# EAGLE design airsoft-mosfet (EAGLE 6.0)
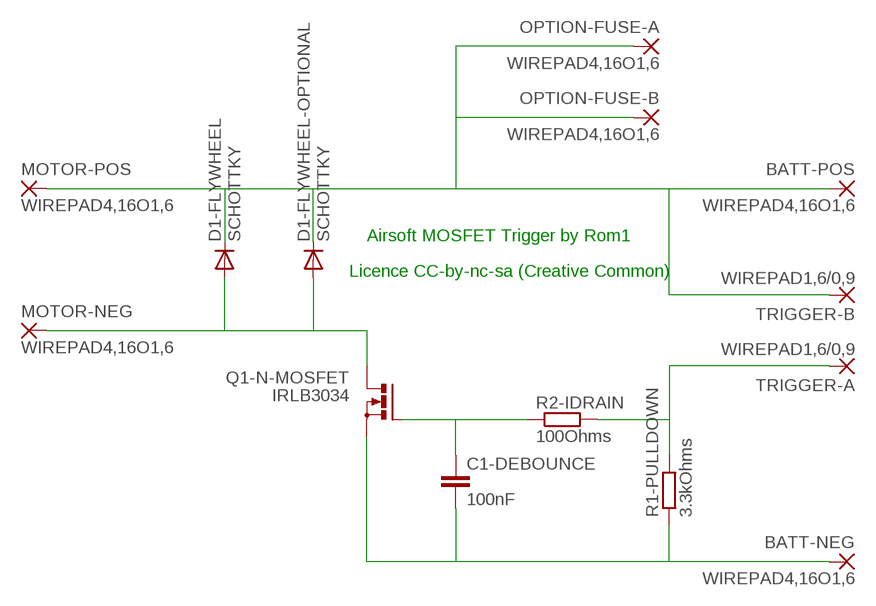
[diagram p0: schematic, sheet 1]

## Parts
BATT-NEG  WIREPAD4,16O1,6  [4,16O1,6]
BATT-POS  WIREPAD4,16O1,6  [4,16O1,6]
C1-DEBOUNCE  100nF  C-EU050-025X075  [C050-025X075]
D1-FLYWHEEL  SCHOTTKY  DIODE-DO201-15  [DO201-15]
D1-FLYWHEEL-OPTIONAL  SCHOTTKY  DIODE-DO201-15  [DO201-15]
MOTOR-NEG  WIREPAD4,16O1,6  [4,16O1,6]
MOTOR-POS  WIREPAD4,16O1,6  [4,16O1,6]
OPTION-FUSE-A  WIREPAD4,16O1,6  [4,16O1,6]
OPTION-FUSE-B  WIREPAD4,16O1,6  [4,16O1,6]
Q1-N-MOSFET  IRLB3034  PMOSFET_NTO220BH  [TO220BH]
R1-PULLDOWN  3.3kOhms  R-EU_0207/10  [0207/10]
R2-IDRAIN  100Ohms  R-EU_0207/10  [0207/10]
TRIGGER-A  WIREPAD1,6/0,9  [1,6/0,9]
TRIGGER-B  WIREPAD1,6/0,9  [1,6/0,9]

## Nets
N$1: BATT-POS.1(P) D1-FLYWHEEL-OPTIONAL.C D1-FLYWHEEL.C MOTOR-POS.1(P) OPTION-FUSE-A.1(P) OPTION-FUSE-B.1(P) TRIGGER-B.1(P)
N$2: D1-FLYWHEEL-OPTIONAL.A D1-FLYWHEEL.A MOTOR-NEG.1(P) Q1-N-MOSFET.D
N$3: C1-DEBOUNCE.1 Q1-N-MOSFET.G R2-IDRAIN.1
N$4: R1-PULLDOWN.2 R2-IDRAIN.2 TRIGGER-A.1(P)
N$5: BATT-NEG.1(P) C1-DEBOUNCE.2 Q1-N-MOSFET.S R1-PULLDOWN.1

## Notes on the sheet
- Airsoft MOSFET Trigger by Rom1
- Licence CC-by-nc-sa (Creative Common)

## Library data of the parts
BATT-NEG BATT-POS MOTOR-NEG MOTOR-POS OPTION-FUSE-A OPTION-FUSE-B TRIGGER-A TRIGGER-B = wirepad:WIREPAD: Wire PAD connect wire on PCB
C1-DEBOUNCE = resistor:C-EU: CAPACITOR, European symbol
D1-FLYWHEEL D1-FLYWHEEL-OPTIONAL = diode:DIODE-: DIODE
Q1-N-MOSFET = transistor-power:PMOSFET_N: Power MOSFET N-Channel
R1-PULLDOWN R2-IDRAIN = resistor:R-EU_: RESISTOR, European symbol

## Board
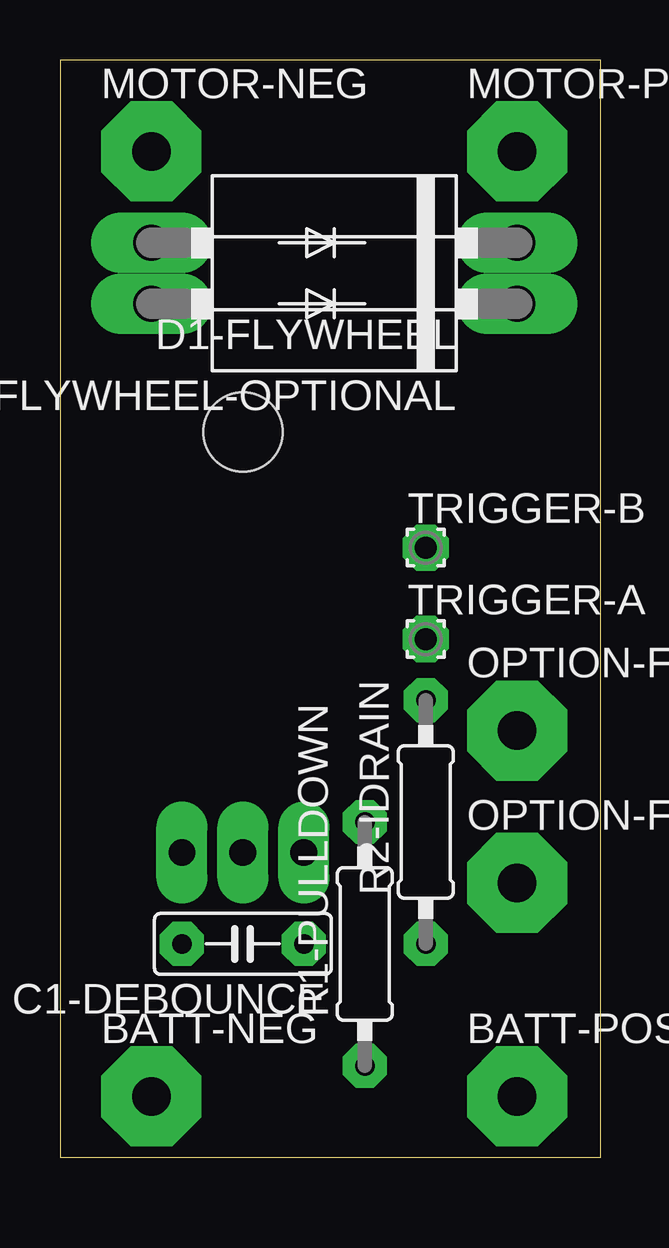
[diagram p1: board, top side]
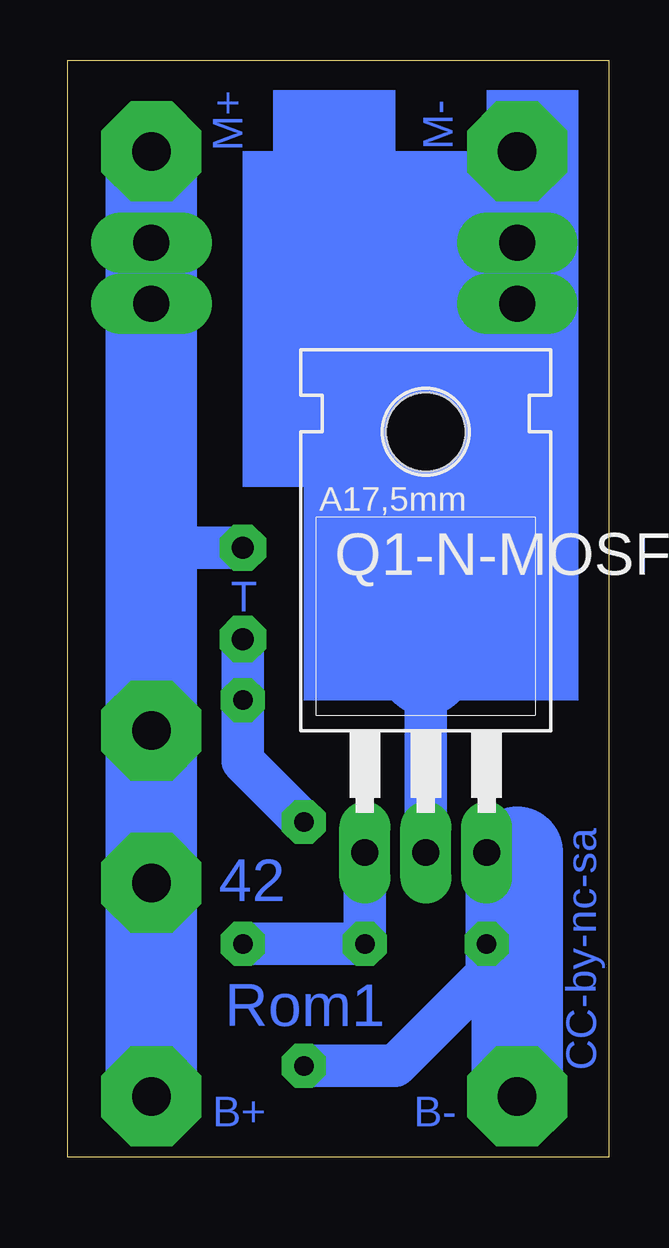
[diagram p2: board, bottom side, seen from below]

Size 22.53 x 45.71 mm. Coordinates in mm from the lower left corner, seen from the top.
Outline: 0,0 22.53,0 22.53,45.71 0,45.71 0,0
Copper layers (1*16): Top 0.035mm / dielectric 1.5mm / Bottom 0.035mm
Design rules: minimum track width 10mil, minimum drill 24mil, track to track 8mil, track to pad 8mil, pad to pad 8mil, via to via 8mil, smd to smd 8mil, copper to edge 40mil, drill to drill 8mil, minimum pad ring 10mil, minimum via ring 8mil, stop-mask expansion 4mil, vias tented up to drill 0mil, thermal gap 10mil

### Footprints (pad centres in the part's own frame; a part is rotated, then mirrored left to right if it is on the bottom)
4,16O1,6 = drill 1.6 pad 4.166 octagon: 1 0,0
C050-025X075 = drill 0.813 octagon: 1 -2.54,0; 2 2.54,0
DO201-15 = drill 1.499 long: A 7.62,0; C -7.62,0
TO220BH = drill 1.118 long: D 0,-6.35; G -2.54,-6.35; S 2.54,-6.35 | hole 3.302: 0,11.176
0207/10 = drill 0.813 octagon: 1 -5.08,0; 2 5.08,0
1,6/0,9 = drill 0.914 pad 1.6 octagon: 1 0,0

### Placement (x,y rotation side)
BATT-NEG  3.81,2.54 0 top
BATT-POS  19.05,2.54 0 top
C1-DEBOUNCE  7.62,8.89 180 top
D1-FLYWHEEL  11.43,38.1 180 top
D1-FLYWHEEL-OPTIONAL  11.43,35.56 180 top
MOTOR-NEG  3.81,41.91 0 top
MOTOR-POS  19.05,41.91 0 top
OPTION-FUSE-A  19.05,11.43 0 top
OPTION-FUSE-B  19.05,17.78 0 top
Q1-N-MOSFET  7.62,19.05 0 bottom
R1-PULLDOWN  12.7,8.89 90 top
R2-IDRAIN  15.24,13.97 90 top
TRIGGER-A  15.24,21.59 0 top
TRIGGER-B  15.24,25.4 0 top

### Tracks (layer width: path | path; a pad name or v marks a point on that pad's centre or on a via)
N$1
  Bottom 1.778: TRIGGER-B.1 19.05,25.4
  Bottom 3.81: MOTOR-POS.1 D1-FLYWHEEL.C D1-FLYWHEEL-OPTIONAL.C 19.05,25.4 OPTION-FUSE-B.1 OPTION-FUSE-A.1 BATT-POS.1
N$2
  Bottom 1.778: Q1-N-MOSFET.D 7.62,20.32
  Bottom 3.81: MOTOR-NEG.1 D1-FLYWHEEL.A D1-FLYWHEEL-OPTIONAL.A 3.81,24.13 7.62,20.32
N$3
  Bottom 1.778: Q1-N-MOSFET.G C1-DEBOUNCE.1 R2-IDRAIN.1
N$4
  Bottom 1.778: TRIGGER-A.1 R2-IDRAIN.2 15.24,16.51 R1-PULLDOWN.2
N$5
  Bottom 1.778: 3.81,12.7 Q1-N-MOSFET.S C1-DEBOUNCE.2 5.08,7.62 8.89,3.81 R1-PULLDOWN.1
  Bottom 3.81: BATT-NEG.1 3.81,12.7
(copper drawn outside any net)
  shapes: Bottom area x4

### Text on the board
Bottom: M+ | M- | T | CC-by-nc-sa | 42 | Rom1 | B- | B+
